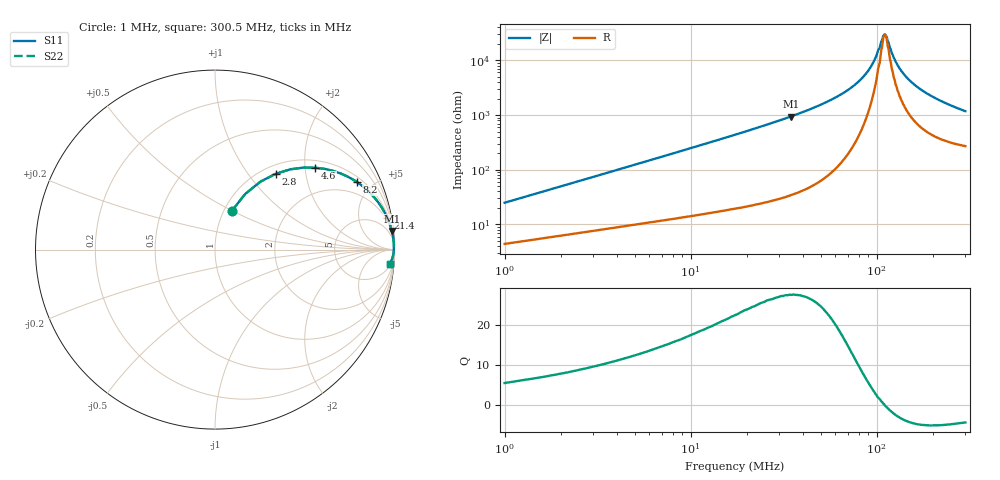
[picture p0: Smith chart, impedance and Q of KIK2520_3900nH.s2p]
!version-2
!date-01.2022
!Series
# MHz S RI R 50
!Freq ReS11 ImS11 ReS21 ImS21 ReS12 ImS12 ReS22 ImS22
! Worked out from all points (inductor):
!   500 points, 1 MHz to 300.5 MHz, reference 50 ohm
!   read as one part in series: L = 3.9 uH near 2.2 MHz
!   highest Q = 27.5 at 34.6 MHz (marker M1), where L = 4.32 uH
!   self-resonance near 111 MHz
!   S11 on the Smith chart (normalised r, x): 1 MHz: 1.09, +0.49; 2.8 MHz: 1.15, +1.37; 4.6 MHz: 1.19, +2.26; 8.2 MHz: 1.25, +4.04; 21.4 MHz: 1, +11; 300.5 MHz: 6, -23
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1  0.0921 0.2131  0.9079 -0.2131  0.9079 -0.2131  0.0921 0.2131
2.8  0.3389 0.4228  0.6611 -0.4228  0.6611 -0.4228  0.3389 0.4228
4.6  0.5574 0.4566  0.4426 -0.4566  0.4426 -0.4566  0.5574 0.4566
8.2  0.7894 0.3775  0.2106 -0.3775  0.2106 -0.3775  0.7894 0.3775
13  0.9013 0.274  0.0987 -0.274  0.0987 -0.274  0.9013 0.274
21.4  0.9608 0.1748  0.0392 -0.1748  0.0392 -0.1748  0.9608 0.1748
34.6  0.9851 0.1043  0.0149 -0.1043  0.0149 -0.1043  0.9851 0.1043
51.4  0.9936 0.0617  0.00639 -0.0617  0.00639 -0.0617  0.9936 0.0617
83.8  0.9971 0.0207  0.00294 -0.0207  0.00294 -0.0207  0.9971 0.0207
94  0.9971 0.0121  0.00291 -0.0121  0.00291 -0.0121  0.9971 0.0121
101  0.997 0.00664  0.00303 -0.00664  0.00303 -0.00664  0.997 0.00664
108.5  0.9967 0.00162  0.00326 -0.00162  0.00326 -0.00162  0.9967 0.00162
111  0.9967 2.85e-05  0.00335 -2.85e-05  0.00335 -2.85e-05  0.9967 2.85e-05
113  0.9966 -0.00114  0.00342 0.00114  0.00342 0.00114  0.9966 -0.00114
121  0.9962 -0.00637  0.00383 0.00637  0.00383 0.00637  0.9962 -0.00637
127  0.9958 -0.00989  0.00418 0.00989  0.00418 0.00989  0.9958 -0.00989
136  0.9952 -0.0149  0.00477 0.0149  0.00477 0.0149  0.9952 -0.0149
151  0.9941 -0.0226  0.00593 0.0226  0.00593 0.0226  0.9941 -0.0226
172  0.9921 -0.0325  0.00788 0.0325  0.00788 0.0325  0.9921 -0.0325
201  0.9889 -0.0446  0.0111 0.0446  0.0111 0.0446  0.9889 -0.0446
251  0.9823 -0.0631  0.0177 0.0631  0.0177 0.0631  0.9823 -0.0631
300.5  0.9745 -0.079  0.0255 0.079  0.0255 0.079  0.9745 -0.079
